| TEXAS INSTRUMENTS INCORPORATED
| Digital Light Processing Group
| IBIS Model of DLP9500
| 0.95_1080p
| This device can be powered at the following Vccs:
|  3.3 volt Vcc
| This file provides unique models under the [Model Selector] for each Vcc.
| For operation at a specific Vcc, select the appropriate model after each
| [Model Selector] keyword.
[IBIS Ver]   3.2
[Comment char]  |_char
[File Name]   dlp9500.ibs
[File Rev]   0.0 | f_die
[Date]   December 21 2012
[Source]   Data created from TI-SPICE at TI-DLP.
[Notes]   The following is an IBIS list for the 0.95_1080p
##notes##|
[Disclaimer] Property of Texas Instruments Incorporated.  Unauthorized
   reproduction and/or distribution is strictly prohibited.
   This product is protected under copyright law.
   Created  2011, (C) Copyright  2011, Texas Instruments
   Incorporated, All Rights Reserved
   UNLESS THERE IS A SIGNED, WRITTEN AGREEMENT TO THE
   CONTRARY, TEXAS INSTRUMENTS (TI) IS PROVIDING THE IBIS
   MODELS  AND WITHOUT ANY WARRANTY, EXPRESSED OR
   IMPLIED.  TI assumes no liability for:
   1) the accuracy of the IBIS models provided to your
   company;
   2) the proper functioning of these IBIS Models in your
   design or for any resulting applications; or
   3) infringement of patents, copyrights or intellectual
   property rights resulting from your use of these IBIS
   models.
   TI provides IBIS Models as a service to our customers.
   You and your company shall not distribute, sell or give
   these models to anyone else without prior written
   permission from TI.
   TI reserves the right to make changes to our products or
   to discontinue any semiconductor product or service
   without notice, and advises our customers to obtain the
   latest version of relevant information to verify, before
   placing orders, that the information being relied on is
   current.
   Please be aware that your receipt and use of the IBIS
   information provided shall serve as acceptance of these
   terms and conditions.  If you do not accept these terms,
   you should return or destroy the IBIS models and any
   other accompanying information immediately.
| Component 0.95_1080p_GKF 355-pin Type-A Device
[Component]   0.95_1080p_GKF
[Manufacturer]   Texas Instruments, Inc.
[Package]
|   typ   min   max
R_pkg   1.59E+00   3.63E-01   3.87E+00
L_pkg   9.02E-09   3.40E-09   2.03E-08
C_pkg   4.02E-12   2.75E-12   6.99E-12
|MBRESET PINS SHOULD BE TIED TO A 250pF CAPACITOR TO GROUND
[Pin]   signal_name   model_name   R_pin   L_pin   C_pin
A1   VSS   GND   1.94E+00   9.75E-09   4.09E-12
A3   VCC   POWER   1.57E+00   1.27E-08   4.07E-12
A5   VCC   POWER   1.89E+00   7.85E-09   4.22E-12
A7   VCC   POWER   1.77E+00   1.30E-08   4.17E-12
A9   VCC   POWER   1.52E+00   1.15E-08   4.16E-12
A11   VCC   POWER   1.57E+00   1.27E-08   4.07E-12
A13   VCC   POWER   1.89E+00   7.85E-09   4.22E-12
A15   D_CP(2)   INPUT_LVDS_BUF  2.19E+00   1.18E-08   3.75E-12
A17   D_CN(2)   INPUT_LVDS_BUF  2.26E+00   1.16E-08   3.81E-12
A19   NO_CONNECT   NC
A21   VCC   POWER   1.57E+00   1.27E-08   4.07E-12
A23   VCC   POWER   1.57E+00   1.27E-08   4.07E-12
A25   VCC   POWER   1.57E+00   1.27E-08   4.07E-12
A27   VCC   POWER   1.57E+00   1.27E-08   4.07E-12
A29   VCC   POWER   1.57E+00   1.27E-08   4.07E-12
AA1   VCC2   POWER   1.57E+00   1.27E-08   4.07E-12
AA3   MBRST(22)   NC
AA5   NO_CONNECT   NC
AA27   MBRST(19)   NC
AA29   MBRST(27)   NC
AA31   VCC   POWER   1.77E+00   1.30E-08   4.17E-12
AB2   VSS   GND   1.94E+00   9.75E-09   4.09E-12
AB4   VSS   GND   1.45E+00   9.13E-09   3.48E-12
AB6   VSS   GND   1.94E+00   9.75E-09   4.09E-12
AB26   VSS   GND   1.74E+00   1.09E-08   2.94E-12
AB28   VSS   GND   1.94E+00   9.75E-09   4.09E-12
AB30   VSS   GND   1.94E+00   9.75E-09   4.09E-12
AC1   VCC   POWER   1.57E+00   1.27E-08   4.07E-12
AC3   SCPDO   TRI_BUF   7.70E-01   7.30E-09   3.87E-12
AC5   NO_CONNECT   NC
AC7   RESERVED_STM   INPUT_BUF   9.46E-01   6.39E-09   4.34E-12
AC9   NO_CONNECT   NC
AC11   NO_CONNECT   NC
AC13   NO_CONNECT   NC
AC15   NO_CONNECT   NC
AC17   NO_CONNECT   NC
AC19   NO_CONNECT   NC
AC21   NO_CONNECT   NC
AC23   NO_CONNECT   NC
AC25   NO_CONNECT   NC
AC27   D_DP(15)   INPUT_LVDS_BUF  1.27E+00   7.50E-09   3.93E-12
AC29   D_DN(15)   INPUT_LVDS_BUF  9.21E-01   5.34E-09   4.60E-12
AC31   VCC   POWER   1.89E+00   7.85E-09   4.22E-12
AD2   SCPDI   INPUT_BUF   6.42E-01   6.98E-09   3.41E-12
AD4   SCPENZ   INPUT_BUF   4.81E-01   5.53E-09   3.63E-12
AD6   VCC1   POWER   1.57E+00   1.27E-08   4.07E-12
AD8   D_BN(1)   INPUT_LVDS_BUF  9.97E-01   6.22E-09   4.78E-12
AD10   D_BP(1)   INPUT_LVDS_BUF  9.21E-01   5.34E-09   4.60E-12
AD12   VCC1   POWER   1.57E+00   1.27E-08   4.07E-12
AD14   D_BP(11)   INPUT_LVDS_BUF  4.05E-01   3.59E-09   3.80E-12
AD16   D_BN(15)   INPUT_LVDS_BUF  6.77E-01   4.29E-09   4.30E-12
AD18   VCC1   POWER   1.57E+00   1.27E-08   4.07E-12
AD20   D_DP(3)   INPUT_LVDS_BUF  4.16E-01   3.48E-09   3.57E-12
AD22   D_DP(7)   INPUT_LVDS_BUF  5.92E-01   3.93E-09   4.02E-12
AD24   VCC1   POWER   1.57E+00   1.27E-08   4.07E-12
AD26   D_DP(13)   INPUT_LVDS_BUF  9.71E-01   5.97E-09   3.66E-12
AD28   D_DN(13)   INPUT_LVDS_BUF  9.88E-01   6.20E-09   3.71E-12
AD30   VSS   GND   1.94E+00   9.75E-09   4.09E-12
AE1   SCPCLK   INPUT_BUF   7.40E-01   8.10E-09   3.49E-12
AE3   D_BN(3)   INPUT_LVDS_BUF  2.30E+00   1.33E-08   5.19E-12
AE5   D_BP(3)   INPUT_LVDS_BUF  2.34E+00   1.21E-08   4.88E-12
AE7   VSS   GND   1.94E+00   9.75E-09   4.09E-12
AE9   D_BP(5)   INPUT_LVDS_BUF  1.09E+00   6.73E-09   4.92E-12
AE11   D_BN(5)   INPUT_LVDS_BUF  1.04E+00   6.06E-09   5.01E-12
AE13   VSS   GND   1.94E+00   9.75E-09   4.09E-12
AE15   D_BN(11)   INPUT_LVDS_BUF  5.02E-01   4.01E-09   3.93E-12
AE17   D_BP(15)   INPUT_LVDS_BUF  4.76E-01   4.42E-09   4.66E-12
AE19   VSS   GND   1.94E+00   9.75E-09   4.09E-12
AE21   D_DN(3)   INPUT_LVDS_BUF  5.11E-01   3.98E-09   3.81E-12
AE23   D_DN(7)   INPUT_LVDS_BUF  6.32E-01   4.66E-09   3.97E-12
AE25   VSS   GND   1.94E+00   9.75E-09   4.09E-12
AE27   D_DN(11)   INPUT_LVDS_BUF  1.56E+00   8.33E-09   3.87E-12
AE29   D_DP(11)   INPUT_LVDS_BUF  1.64E+00   8.36E-09   3.90E-12
AE31   VCC   POWER   1.57E+00   1.27E-08   4.07E-12
AF2   SCTRL_BP   INPUT_LVDS_BUF  3.58E+00   1.72E-08   5.73E-12
AF4   SCTRL_BN   INPUT_LVDS_BUF  3.55E+00   1.68E-08   5.59E-12
AF6   VSS   GND   1.94E+00   9.75E-09   4.09E-12
AF8   D_BP(7)   INPUT_LVDS_BUF  1.51E+00   8.13E-09   5.50E-12
AF10   D_BN(7)   INPUT_LVDS_BUF  1.49E+00   7.98E-09   5.41E-12
AF12   VSS   GND   1.94E+00   9.75E-09   4.09E-12
AF14   D_BN(13)   INPUT_LVDS_BUF  8.38E-01   5.57E-09   3.97E-12
AF16   D_BP(13)   INPUT_LVDS_BUF  7.75E-01   4.88E-09   3.97E-12
AF18   VSS   GND   1.94E+00   9.75E-09   4.09E-12
AF20   D_DN(5)   INPUT_LVDS_BUF  9.15E-01   5.80E-09   3.86E-12
AF22   D_DP(5)   INPUT_LVDS_BUF  8.28E-01   5.50E-09   4.02E-12
AF24   VSS   GND   1.94E+00   9.75E-09   4.09E-12
AF26   D_DP(9)   INPUT_LVDS_BUF  1.50E+00   8.34E-09   4.15E-12
AF28   D_DN(9)   INPUT_LVDS_BUF  1.57E+00   8.66E-09   4.24E-12
AF30   VSS   GND   1.94E+00   9.75E-09   4.09E-12
AG1   VCC   POWER   1.89E+00   7.85E-09   4.22E-12
AG3   D_BP(9)   INPUT_LVDS_BUF  3.56E+00   1.77E-08   6.16E-12
AG5   D_BN(9)   INPUT_LVDS_BUF  3.50E+00   1.71E-08   6.07E-12
AG7   VSS   GND   1.94E+00   9.75E-09   4.09E-12
AG9   D_BN(4)   INPUT_LVDS_BUF  1.17E+00   6.77E-09   4.44E-12
AG11   D_BP(4)   INPUT_LVDS_BUF  1.49E+00   1.50E-08   6.54E-12
AG13   VSS   GND   1.94E+00   9.75E-09   4.09E-12
AG15   D_DN(1)   INPUT_LVDS_BUF  1.76E+00   9.70E-09   4.39E-12
AG17   D_DP(1)   INPUT_LVDS_BUF  1.70E+00   9.04E-09   4.27E-12
AG19   VSS   GND   1.94E+00   9.75E-09   4.09E-12
AG21   SCTRL_DP   INPUT_LVDS_BUF  1.20E+00   7.15E-09   3.86E-12
AG23   SCTRL_DN   INPUT_LVDS_BUF  1.26E+00   7.23E-09   4.04E-12
AG25   VSS   GND   1.94E+00   9.75E-09   4.09E-12
AG27   D_DP(14)   INPUT_LVDS_BUF  1.49E+00   8.33E-09   3.91E-12
AG29   D_DN(14)   INPUT_LVDS_BUF  1.54E+00   8.40E-09   4.03E-12
AG31   VCC   POWER   1.89E+00   7.85E-09   4.22E-12
AH2   D_BN(0)   INPUT_LVDS_BUF  2.65E+00   1.35E-08   4.62E-12
AH4   D_BP(0)   INPUT_LVDS_BUF  2.56E+00   1.32E-08   4.67E-12
AH6   VSS   GND   1.94E+00   9.75E-09   4.09E-12
AH8   D_BP(6)   INPUT_LVDS_BUF  1.49E+00   8.61E-09   4.27E-12
AH10   D_BN(6)   INPUT_LVDS_BUF  1.59E+00   8.48E-09   4.05E-12
AH12   VSS   GND   1.94E+00   9.75E-09   4.09E-12
AH14   D_BN(12)   INPUT_LVDS_BUF  1.03E+00   6.27E-09   3.41E-12
AH16   D_BP(12)   INPUT_LVDS_BUF  9.64E-01   5.97E-09   3.39E-12
AH18   VSS   GND   1.94E+00   9.75E-09   4.09E-12
AH20   D_DP(6)   INPUT_LVDS_BUF  9.94E-01   6.21E-09   3.38E-12
AH22   D_DN(6)   INPUT_LVDS_BUF  1.08E+00   6.62E-09   3.56E-12
AH24   VSS   GND   1.94E+00   9.75E-09   4.09E-12
AH26   D_DN(12)   INPUT_LVDS_BUF  1.38E+00   8.01E-09   3.61E-12
AH28   D_DP(12)   INPUT_LVDS_BUF  1.28E+00   8.02E-09   3.82E-12
AH30   VSS   GND   1.94E+00   9.75E-09   4.09E-12
AJ1   VSS   GND   1.94E+00   9.75E-09   4.09E-12
AJ3   D_BP(2)   INPUT_LVDS_BUF  2.54E+00   1.32E-08   4.49E-12
AJ5   D_BN(2)   INPUT_LVDS_BUF  2.59E+00   1.34E-08   4.44E-12
AJ7   VSS   GND   1.94E+00   9.75E-09   4.09E-12
AJ9   DCLK_BP   INPUT_LVDS_BUF  1.59E+00   9.22E-09   3.76E-12
AJ11   DCLK_BN   INPUT_LVDS_BUF  1.66E+00   9.18E-09   3.71E-12
AJ13   VSS   GND   1.94E+00   9.75E-09   4.09E-12
AJ15   D_BP(14)   INPUT_LVDS_BUF  1.21E+00   7.37E-09   3.41E-12
AJ17   D_BN(14)   INPUT_LVDS_BUF  1.30E+00   7.61E-09   3.44E-12
AJ19   VSS   GND   1.94E+00   9.75E-09   4.09E-12
AJ21   DCLK_DP   INPUT_LVDS_BUF  1.21E+00   7.23E-09   3.41E-12
AJ23   DCLK_DN   INPUT_LVDS_BUF  1.26E+00   7.86E-09   3.38E-12
AJ25   VSS   GND   1.94E+00   9.75E-09   4.09E-12
AJ27   D_DP(10)   INPUT_LVDS_BUF  2.07E+00   1.09E-08   4.45E-12
AJ29   D_DN(10)   INPUT_LVDS_BUF  2.14E+00   1.13E-08   4.25E-12
AJ31   VCC   POWER   1.89E+00   7.85E-09   4.22E-12
AK2   VCC   POWER   1.89E+00   7.85E-09   4.22E-12
AK4   NO_CONNECT   NC
AK6   VSS   GND   1.94E+00   9.75E-09   4.09E-12
AK8   D_BN(8)   INPUT_LVDS_BUF  2.40E+00   1.23E-08   4.40E-12
AK10   D_BP(8)   INPUT_LVDS_BUF  2.28E+00   1.16E-08   4.31E-12
AK12   VSS   GND   1.94E+00   9.75E-09   4.09E-12
AK14   D_DN(0)   INPUT_LVDS_BUF  2.49E+00   1.27E-08   4.25E-12
AK16   D_DP(0)   INPUT_LVDS_BUF  2.41E+00   1.26E-08   4.22E-12
AK18   VSS   GND   1.94E+00   9.75E-09   4.09E-12
AK20   D_DN(4)   INPUT_LVDS_BUF  1.78E+00   9.43E-09   3.73E-12
AK22   D_DP(4)   INPUT_LVDS_BUF  1.67E+00   9.13E-09   3.70E-12
AK24   NO_CONNECT   NC
AK26   D_DN(8)   INPUT_LVDS_BUF  2.23E+00   1.15E-08   3.98E-12
AK28   D_DP(8)   INPUT_LVDS_BUF  2.14E+00   1.17E-08   4.10E-12
AK30   VCC   POWER   1.89E+00   7.85E-09   4.22E-12
AL3   VCC   POWER   1.89E+00   7.85E-09   4.22E-12
AL5   VCC   POWER   1.89E+00   7.85E-09   4.22E-12
AL7   VCC   POWER   1.89E+00   7.85E-09   4.22E-12
AL9   D_BP(10)   INPUT_LVDS_BUF  2.23E+00   1.18E-08   3.68E-12
AL11   D_BN(10)   INPUT_LVDS_BUF  2.28E+00   1.21E-08   3.84E-12
AL13   NO_CONNECT   NC
AL15   D_DP(2)   INPUT_LVDS_BUF  2.34E+00   1.28E-08   4.00E-12
AL17   D_DN(2)   INPUT_LVDS_BUF  2.42E+00   1.20E-08   3.90E-12
AL19   VCC   POWER   1.57E+00   1.27E-08   4.07E-12
AL21   VCC   POWER   1.57E+00   1.27E-08   4.07E-12
AL23   VCC   POWER   1.57E+00   1.27E-08   4.07E-12
AL25   VCC   POWER   1.57E+00   1.27E-08   4.07E-12
AL27   VCC   POWER   1.57E+00   1.27E-08   4.07E-12
AL29   VSS   GND   1.58E+00   8.55E-09   3.17E-12
B2   VCC   POWER   1.57E+00   1.27E-08   4.07E-12
B4   PWRDNZ   INPUT_BUF   1.14E+00   1.10E-08   4.69E-12
B6   NO_CONNECT   NC
B8   D_AP(10)   INPUT_LVDS_BUF  2.29E+00   1.18E-08   3.93E-12
B10   D_AN(10)   INPUT_LVDS_BUF  2.28E+00   1.16E-08   3.82E-12
B12   VSS   GND   1.58E+00   8.55E-09   3.17E-12
B14   D_CN(0)   INPUT_LVDS_BUF  2.34E+00   1.21E-08   4.23E-12
B16   D_CP(0)   INPUT_LVDS_BUF  2.25E+00   1.17E-08   4.24E-12
B18   VSS   GND   1.58E+00   8.55E-09   3.17E-12
B20   D_CN(4)   INPUT_LVDS_BUF  1.80E+00   9.49E-09   3.75E-12
B22   D_CP(4)   INPUT_LVDS_BUF  1.69E+00   9.74E-09   3.69E-12
B24   VSS   GND   1.58E+00   8.55E-09   3.17E-12
B26   D_CN(8)   INPUT_LVDS_BUF  2.24E+00   1.15E-08   3.90E-12
B28   D_CP(8)   INPUT_LVDS_BUF  2.14E+00   1.16E-08   4.14E-12
B30   VSS   GND   1.58E+00   8.55E-09   3.17E-12
C1   VCC   POWER   1.89E+00   7.85E-09   4.22E-12
C3   RESERVED_AE   INPUT_BUF   1.02E+00   8.78E-09   4.42E-12
C5   NO_CONNECT   NC
C7   VSS   GND   1.75E+00   7.30E-09   3.10E-12
C9   D_AN(8)   INPUT_LVDS_BUF  1.77E+00   9.51E-09   4.33E-12
C11   D_AP(8)   INPUT_LVDS_BUF  1.61E+00   8.73E-09   4.27E-12
C13   VSS   GND   1.75E+00   7.30E-09   3.10E-12
C15   D_AP(14)   INPUT_LVDS_BUF  1.20E+00   7.14E-09   3.59E-12
C17   D_AN(14)   INPUT_LVDS_BUF  1.28E+00   7.33E-09   3.32E-12
C19   VSS   GND   1.75E+00   7.30E-09   3.10E-12
C21   DCLK_CP   INPUT_LVDS_BUF  1.21E+00   7.36E-09   3.35E-12
C23   DCLK_CN   INPUT_LVDS_BUF  1.27E+00   7.49E-09   3.54E-12
C25   VSS   GND   1.75E+00   7.30E-09   3.10E-12
C27   D_CP(10)   INPUT_LVDS_BUF  2.08E+00   1.12E-08   4.28E-12
C29   D_CN(10)   INPUT_LVDS_BUF  2.14E+00   1.12E-08   4.24E-12
C31   VCC   POWER   1.74E+00   9.67E-09   3.96E-12
D2   D_AN(4)   INPUT_LVDS_BUF  2.96E+00   1.45E-08   5.37E-12
D4   D_AP(4)   INPUT_LVDS_BUF  2.87E+00   1.42E-08   5.25E-12
D6   VSS   GND   1.75E+00   7.30E-09   3.10E-12
D8   DCLK_AP   INPUT_LVDS_BUF  1.59E+00   8.91E-09   4.27E-12
D10   DCLK_AN   INPUT_LVDS_BUF  1.66E+00   8.80E-09   4.38E-12
D12   VSS   GND   1.75E+00   7.30E-09   3.10E-12
D14   D_AN(12)   INPUT_LVDS_BUF  1.03E+00   6.24E-09   3.73E-12
D16   D_AP(12)   INPUT_LVDS_BUF  9.62E-01   6.16E-09   3.50E-12
D18   VSS   GND   1.75E+00   7.30E-09   3.10E-12
D20   D_CP(6)   INPUT_LVDS_BUF  9.92E-01   6.24E-09   3.58E-12
D22   D_CN(6)   INPUT_LVDS_BUF  1.07E+00   6.64E-09   3.47E-12
D24   VSS   GND   1.75E+00   7.30E-09   3.10E-12
D26   D_CN(12)   INPUT_LVDS_BUF  1.39E+00   7.92E-09   3.70E-12
D28   D_CP(12)   INPUT_LVDS_BUF  1.27E+00   8.03E-09   3.62E-12
D30   VSS   GND   1.75E+00   7.30E-09   3.10E-12
E1   VSS   GND   1.75E+00   7.30E-09   3.10E-12
E3   D_AP(2)   INPUT_LVDS_BUF  2.27E+00   1.16E-08   4.75E-12
E5   D_AN(2)   INPUT_LVDS_BUF  2.35E+00   1.19E-08   4.90E-12
E7   VSS   GND   1.75E+00   7.30E-09   3.10E-12
E9   D_AP(6)   INPUT_LVDS_BUF  1.14E+00   6.88E-09   4.67E-12
E11   D_AN(6)   INPUT_LVDS_BUF  1.21E+00   6.72E-09   4.64E-12
E13   VSS   GND   1.75E+00   7.30E-09   3.10E-12
E15   D_CN(1)   INPUT_LVDS_BUF  1.76E+00   9.48E-09   4.27E-12
E17   D_CP(1)   INPUT_LVDS_BUF  1.71E+00   9.38E-09   4.18E-12
E19   VSS   GND   1.75E+00   7.30E-09   3.10E-12
E21   SCTRL_CP   INPUT_LVDS_BUF  1.20E+00   7.16E-09   4.06E-12
E23   SCTRL_CN   INPUT_LVDS_BUF  1.23E+00   6.93E-09   3.83E-12
E25   VSS   GND   1.75E+00   7.30E-09   3.10E-12
E27   D_CP(14)   INPUT_LVDS_BUF  1.49E+00   8.37E-09   4.24E-12
E29   D_CN(14)   INPUT_LVDS_BUF  1.54E+00   8.55E-09   4.17E-12
E31   VCC   POWER   1.74E+00   9.67E-09   3.96E-12
F2   D_AN(0)   INPUT_LVDS_BUF  2.56E+00   1.27E-08   4.54E-12
F4   D_AP(0)   INPUT_LVDS_BUF  2.46E+00   1.23E-08   4.68E-12
F6   VSS   GND   1.77E+00   1.14E-08   2.83E-12
F8   D_AN(7)   INPUT_LVDS_BUF  1.58E+00   8.68E-09   4.34E-12
F10   D_AP(7)   INPUT_LVDS_BUF  1.60E+00   7.82E-09   4.29E-12
F12   VSS   GND   1.77E+00   1.14E-08   2.83E-12
F14   D_AN(13)   INPUT_LVDS_BUF  8.14E-01   5.53E-09   3.96E-12
F16   D_AP(13)   INPUT_LVDS_BUF  7.63E-01   4.80E-09   3.89E-12
F18   VSS   GND   1.77E+00   1.14E-08   2.83E-12
F20   D_CN(5)   INPUT_LVDS_BUF  9.12E-01   5.79E-09   3.87E-12
F22   D_CP(5)   INPUT_LVDS_BUF  8.02E-01   5.20E-09   4.06E-12
F24   VSS   GND   1.77E+00   1.14E-08   2.83E-12
F26   D_CP(9)   INPUT_LVDS_BUF  1.49E+00   8.20E-09   4.25E-12
F28   D_CN(9)   INPUT_LVDS_BUF  1.57E+00   8.61E-09   4.30E-12
F30   VSS   GND   1.63E+00   1.09E-08   4.27E-12
G1   MODE_B   INPUT_BUF   1.11E+00   1.13E-08   4.63E-12
G3   D_AN(5)   INPUT_LVDS_BUF  2.75E+00   1.49E-08   5.40E-12
G5   D_AP(5)   INPUT_LVDS_BUF  2.66E+00   1.41E-08   5.22E-12
G7   VSS   GND   1.77E+00   1.14E-08   2.83E-12
G9   D_AN(3)   INPUT_LVDS_BUF  8.77E-01   5.88E-09   4.73E-12
G11   D_AP(3)   INPUT_LVDS_BUF  7.86E-01   4.82E-09   4.44E-12
G13   VSS   GND   1.77E+00   1.14E-08   2.83E-12
G15   D_AN(11)   INPUT_LVDS_BUF  4.99E-01   3.86E-09   3.72E-12
G17   D_AP(15)   INPUT_LVDS_BUF  3.63E-01   3.81E-09   4.10E-12
G19   VSS   GND   1.77E+00   1.14E-08   2.83E-12
G21   D_CN(3)   INPUT_LVDS_BUF  4.74E-01   3.76E-09   3.87E-12
G23   D_CN(7)   INPUT_LVDS_BUF  6.34E-01   4.52E-09   4.46E-12
G25   VSS   GND   1.77E+00   1.14E-08   2.83E-12
G27   D_CN(11)   INPUT_LVDS_BUF  1.59E+00   8.49E-09   3.88E-12
G29   D_CP(11)   INPUT_LVDS_BUF  1.66E+00   8.77E-09   3.99E-12
G31   VCC   POWER   1.74E+00   9.67E-09   3.96E-12
H2   D_AN(9)   INPUT_LVDS_BUF  3.87E+00   2.03E-08   5.48E-12
H4   D_AP(9)   INPUT_LVDS_BUF  3.81E+00   2.03E-08   5.91E-12
H6   VCC1   POWER   1.74E+00   9.67E-09   3.96E-12
H8   D_AN(1)   INPUT_LVDS_BUF  8.74E-01   5.94E-09   4.70E-12
H10   D_AP(1)   INPUT_LVDS_BUF  7.90E-01   4.93E-09   4.44E-12
H12   VCC1   POWER   1.74E+00   9.67E-09   3.96E-12
H14   D_AP(11)   INPUT_LVDS_BUF  4.17E-01   3.59E-09   3.72E-12
H16   D_AN(15)   INPUT_LVDS_BUF  4.64E-01   3.69E-09   4.09E-12
H18   VCC1   POWER   1.74E+00   9.67E-09   3.96E-12
H20   D_CP(3)   INPUT_LVDS_BUF  4.17E-01   3.40E-09   4.09E-12
H22   D_CP(7)   INPUT_LVDS_BUF  6.02E-01   3.93E-09   4.12E-12
H24   VCC1   POWER   1.74E+00   9.67E-09   3.96E-12
H26   D_CP(13)   INPUT_LVDS_BUF  9.77E-01   5.88E-09   3.59E-12
H28   D_CN(13)   INPUT_LVDS_BUF  9.85E-01   6.57E-09   3.61E-12
H30   NO_CONNECT   NC
J1   MODE_A   INPUT_BUF   1.02E+00   1.07E-08   4.54E-12
J3   SCTRL_AN   INPUT_LVDS_BUF  3.04E+00   1.68E-08   5.72E-12
J5   SCTRL_AP   INPUT_LVDS_BUF  2.99E+00   1.62E-08   5.67E-12
J7   RESERVED_FC   INPUT_BUF   4.26E-01   4.47E-09   3.77E-12
J9   RESERVED_FD   INPUT_BUF   4.57E-01   4.91E-09   4.39E-12
J11   RESERVED_PFE   INPUT_BUF   9.44E-01   9.09E-09   5.36E-12
J13   NO_CONNECT   NC
J15   NO_CONNECT   NC
J17   NO_CONNECT   NC
J19   NO_CONNECT   NC
J21   NO_CONNECT   NC
J23   NO_CONNECT   NC
J25   NO_CONNECT   NC
J27   D_CP(15)   INPUT_LVDS_BUF  1.25E+00   7.01E-09   3.73E-12
J29   D_CN(15)   INPUT_LVDS_BUF  1.26E+00   7.28E-09   3.86E-12
J31   VCC   POWER   1.74E+00   9.67E-09   3.96E-12
K2   VCC   POWER   1.74E+00   9.67E-09   3.96E-12
K4   VSS   GND   1.31E+00   5.77E-09   2.75E-12
K6   VSS   GND   1.31E+00   5.77E-09   2.75E-12
K26   VSS   GND   1.31E+00   5.77E-09   2.75E-12
K28   VSS   GND   1.31E+00   5.77E-09   2.75E-12
K30   VSS   GND   1.31E+00   5.77E-09   2.75E-12
L1   VCC2   POWER   1.74E+00   9.67E-09   3.96E-12
L3   MBRST(4)   NC
L5   MBRST(0)   NC
L27   MBRST(13)   NC
L29   MBRST(9)   NC
L31   VCC   POWER   1.74E+00   9.67E-09   3.96E-12
M2   VSS   GND   1.31E+00   5.77E-09   2.75E-12
M4   MBRST(8)   NC
M6   VCC1   POWER   1.74E+00   9.67E-09   3.96E-12
M26   VCC1   POWER   1.74E+00   9.67E-09   3.96E-12
M28   MBRST(1)   NC
M30   VSS   GND   1.31E+00   5.77E-09   2.75E-12
N1   VCC2   POWER   1.74E+00   9.67E-09   3.96E-12
N3   MBRST(12)   NC
N5   VSS   GND   1.31E+00   5.77E-09   2.75E-12
N27   VSS   GND   1.31E+00   5.77E-09   2.75E-12
N29   MBRST(11)   NC
N31   VCC   POWER   1.74E+00   9.67E-09   3.96E-12
P2   MBRST(6)   NC
P4   MBRST(2)   NC
P6   VCC1   POWER   1.74E+00   9.67E-09   3.96E-12
P26   VCC1   POWER   1.74E+00   9.67E-09   3.96E-12
P28   MBRST(5)   NC
P30   MBRST(3)   NC
R1   VCC2   POWER   1.74E+00   9.67E-09   3.96E-12
R3   MBRST(14)   NC
R5   VSS   GND   1.31E+00   5.77E-09   2.75E-12
R27   NO_CONNECT   NC
R29   MBRST(17)   NC
R31   VCC   POWER   1.74E+00   9.67E-09   3.96E-12
T2   VSS   GND   1.31E+00   5.77E-09   2.75E-12
T4   MBRST(10)   NC
T6   VCC1   POWER   1.74E+00   9.67E-09   3.96E-12
T26   VCC1   POWER   1.74E+00   9.67E-09   3.96E-12
T28   MBRST(7)   NC
T30   VSS   GND   1.31E+00   5.77E-09   2.75E-12
U1   VCC2   POWER   1.74E+00   9.67E-09   3.96E-12
U3   MBRST(28)   NC
U5   MBRST(24)   NC
U27   VSS   GND   1.31E+00   5.77E-09   2.75E-12
U29   MBRST(25)   NC
U31   VCC   POWER   1.74E+00   9.67E-09   3.96E-12
V2   VSS   GND   1.31E+00   5.77E-09   2.75E-12
V4   MBRST(16)   NC
V6   VCC1   POWER   1.74E+00   9.67E-09   3.96E-12
V26   VCC1   POWER   1.74E+00   9.67E-09   3.96E-12
V28   MBRST(15)   NC
V30   VSS   GND   1.31E+00   5.77E-09   2.75E-12
W1   VCC2   POWER   1.74E+00   9.67E-09   3.96E-12
W3   MBRST(20)   NC
W5   VSS   GND   1.31E+00   5.77E-09   2.75E-12
W27   MBRST(21)   NC
W29   MBRST(23)   NC
W31   VCC   POWER   1.74E+00   9.67E-09   3.96E-12
Y2   MBRST(26)   NC
Y4   MBRST(18)   NC
Y6   VCC1   POWER   1.74E+00   9.67E-09   3.96E-12
Y26   VCC1   POWER   1.74E+00   9.67E-09   3.96E-12
Y28   VSS   GND   1.31E+00   5.77E-09   2.75E-12
Y30   MBRST(29)   NC
| NOTE:  The [Diff Pin] section is commented out because the ibischk3 program
|   currently flags it as an Error when it shouldn't
| [Diff Pin]  inv_pin   vdiff   tdelay_typ
| F4   F2   400mv   NA
| H10   H8   400mv   NA
| E3   E5   400mv   NA
| G11   G9   400mv   NA
| D4   D2   400mv   NA
| G5   G3   400mv   NA
| E9   E11   400mv   NA
| F10   F8   400mv   NA
| C11   C9   400mv   NA
| H4   H2   400mv   NA
| B8   B10   400mv   NA
| H14   G15   400mv   NA
| D16   D14   400mv   NA
| F16   F14   400mv   NA
| C15   C17   400mv   NA
| H16   H16   400mv   NA
| D8   D10   400mv   NA
| J5   J3   400mv   NA
| AH4   AH2   400mv   NA
| AD10   AD8   400mv   NA
| AJ3   AJ5   400mv   NA
| AE5   AE3   400mv   NA
| AG11   AG9   400mv   NA
| AE9   AE11   400mv   NA
| AH8   AH10   400mv   NA
| AF8   AF10   400mv   NA
| AK10   AK8   400mv   NA
| AG3   AG5   400mv   NA
| AL9   AL11   400mv   NA
| AD14   AE15   400mv   NA
| AH16   AH14   400mv   NA
| AF16   AF14   400mv   NA
| AJ15   AJ17   400mv   NA
| AE17   AD16   400mv   NA
| AJ9   AJ11   400mv   NA
| AF2   AF4   400mv   NA
| B16   B14   400mv   NA
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[Model Selector]   INPUT_LVDS_BUF
INPUT_LVDS_BUF_33   3.3 volt Vcc
| Model INPUT_BUF
[Model Selector]   INPUT_BUF
INPUT_BUF_33   3.3 volt Vcc
| Model OUTPUT_BUF
[Model Selector]   OUTPUT_BUF
OUTPUT_BUF_33   3.3 volt Vcc
| Model TRI_BUF
[Model Selector]   TRI_BUF
TRI_BUF_33   3.3 volt Vcc
| Models and submodels in the file (4): INPUT_LVDS_BUF_33 (Input), INPUT_BUF_33 (Input), OUTPUT_BUF_33 (Output), TRI_BUF_33 (3-state)
